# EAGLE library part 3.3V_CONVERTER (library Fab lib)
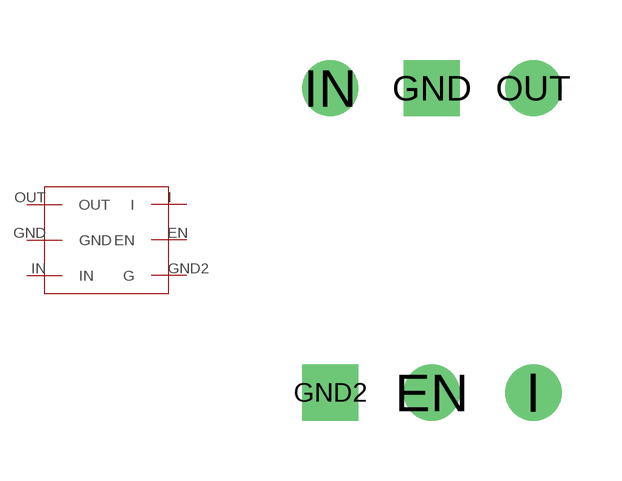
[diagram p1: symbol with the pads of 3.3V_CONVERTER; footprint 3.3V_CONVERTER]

Designator prefix -

## 3.3V_CONVERTER  [3.3V_CONVERTER]
EN  EN  in
GND  GND  pwr
GND2  G  pwr
I  I  in
IN  IN  in
OUT  OUT  out

## Footprint 3.3V_CONVERTER (pad centres in mm)
drill 0.9: EN 0,-5.08; I 2.54,-5.08; IN -2.54,2.54; OUT 2.54,2.54
drill 0.9 square: GND 0,2.54; GND2 -2.54,-5.08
